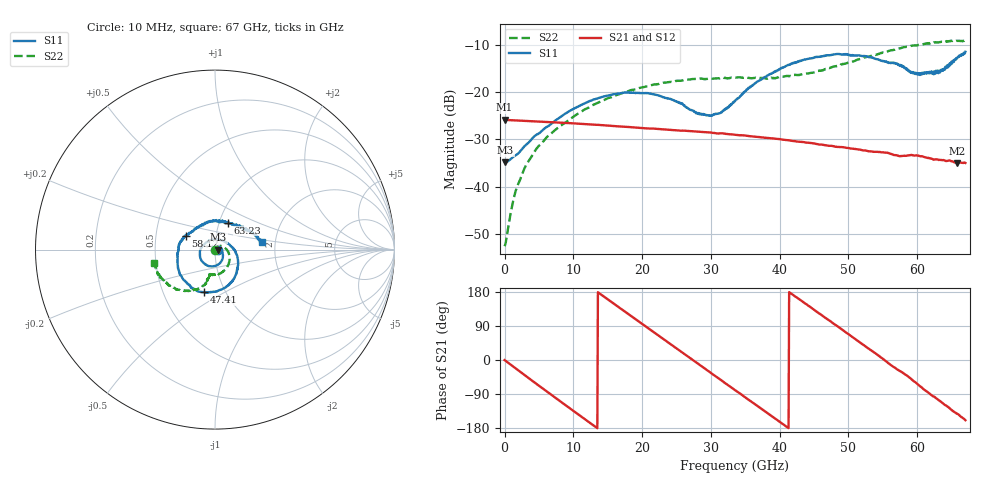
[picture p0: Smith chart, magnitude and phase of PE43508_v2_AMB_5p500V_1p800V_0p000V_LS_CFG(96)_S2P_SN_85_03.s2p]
!Keysight Technologies,N5227A,US51270237,A.10.43.00
!Date: Wednesday, August 22, 2018 17:16:41
!Correction: S11(Full 2 Port(1,3))
!S31(Full 2 Port(1,3))
!S13(Full 2 Port(1,3))
!S33(Full 2 Port(1,3))
!S2P File: Measurements: S11, S31, S13, S33:
# Hz S  dB  R 50
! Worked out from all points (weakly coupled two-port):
!   801 points, 10 MHz to 67 GHz, reference 50 ohm
!   highest |S21| = -25.88 dB at 10 MHz (marker M1); lowest = -35.0 dB at 65.83 GHz (marker M2)
!   lowest |S11| = -34.9 dB at 93.74 MHz (marker M3), VSWR 1.04, Z = 51.8 + j0.0124 ohm
!   |S11| at or under -10 dB: start of sweep to end of sweep
!   |S22| runs from -52.5 to -9.1 dB; largest |S21 - S12| = 0.00025
!   S11 on the Smith chart (normalised r, x): 10 MHz: 1.04, -0.00; 47.41 GHz: 0.79, -0.40; 58.12 GHz: 0.71, +0.11; 63.23 GHz: 1.10, +0.34; 67 GHz: 1.70, +0.15
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1e7  -34.77 -1.1  -25.88 -0.3  -25.88 -0.2  -52.52 -176.6
9.37375e7  -34.86 0.4  -25.89 -1.4  -25.90 -1.4  -52.21 165.8
1.517275e9  -33.46 4.4  -25.99 -21.0  -25.99 -21.0  -41.40 85.1
3.275762e9  -30.99 -0.0  -26.11 -44.8  -26.11 -44.8  -35.07 62.6
6.206575e9  -27.35 -18.5  -26.31 -84.0  -26.31 -83.9  -29.48 39.5
1.123082e10  -22.66 -60.6  -26.73 -150.4  -26.74 -150.4  -24.09 2.4
1.74274e10  -20.15 -111.6  -27.33 128.7  -27.33 128.7  -20.08 -34.5
2.236791e10  -20.73 -155.1  -27.83 64.6  -27.83 64.6  -18.31 -59.1
2.973681e10  -24.98 96.3  -28.54 -30.5  -28.54 -30.6  -17.16 -85.8
3.132782e10  -24.46 63.3  -28.73 -50.7  -28.73 -50.8  -17.10 -90.4
3.3505e10  -21.96 24.0  -29.04 -79.5  -29.04 -79.5  -16.98 -95.5
3.643581e10  -18.16 -13.1  -29.43 -117.0  -29.43 -117.1  -17.03 -100.0
3.88642e10  -16.12 -35.5  -29.78 -148.2  -29.79 -148.2  -17.08 -101.0
4.472582e10  -12.88 -83.9  -30.80 136.0  -30.79 136.0  -15.96 -102.6
4.740542e10  -12.23 -104.7  -31.35 101.8  -31.33 101.8  -14.87 -104.8
5.234594e10  -12.42 -144.1  -32.34 37.6  -32.31 37.6  -12.75 -111.4
5.586291e10  -13.91 -179.4  -32.90 -9.3  -32.87 -9.8  -11.34 -121.8
5.812382e10  -14.98 155.2  -33.48 -36.6  -33.47 -36.9  -10.55 -129.3
6.004979e10  -16.01 122.2  -33.40 -63.7  -33.41 -64.1  -10.16 -136.8
6.323181e10  -15.56 64.4  -34.31 -107.3  -34.36 -107.8  -9.50 -150.4
6.582768e10  -12.75 24.1  -35.00 -142.0  -35.07 -142.3  -9.24 -160.9
6.7e10  -11.53 8.8  -34.98 -158.9  -35.08 -159.0  -9.18 -167.4
